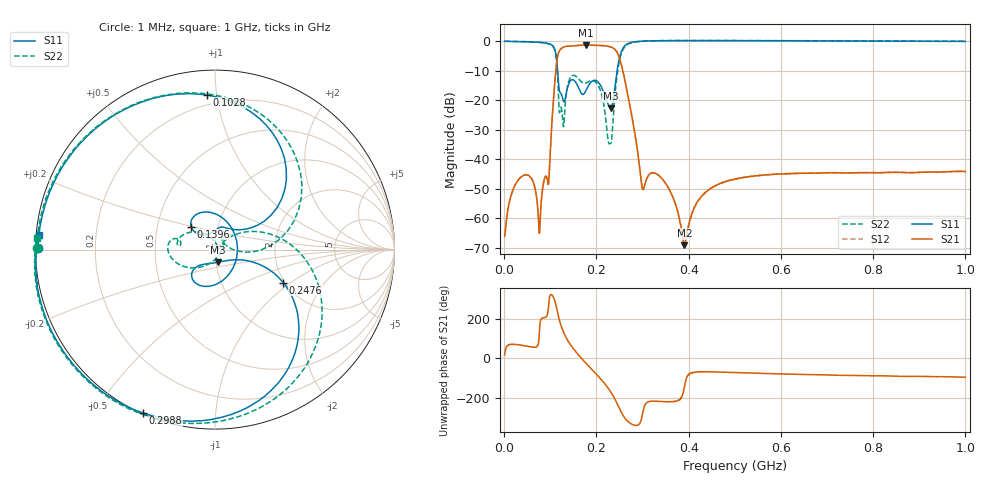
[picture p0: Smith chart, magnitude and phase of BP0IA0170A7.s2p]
!Agilent Technologies,E8358A,US41080443,A.07.50.56
!Agilent E8358A: A.07.50.56
!Date: Tuesday, October 31, 2017 22:14:20
!Correction: S11(Full 2 Port(1,2))
!S21(Full 2 Port(1,2))
!S12(Full 2 Port(1,2))
!S22(Full 2 Port(1,2))
!S2P File: Measurements: S11, S21, S12, S22:
# Hz S  dB  R 50
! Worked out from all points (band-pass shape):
!   1601 points, 1 MHz to 1 GHz, reference 50 ohm
!   highest |S21| = -1.31 dB at 177.7 MHz (marker M1); lowest = -69.2 dB at 390.6 MHz (marker M2)
!   |S21| within 3 dB of the highest: 117.2 MHz to 246.4 MHz (129.2 MHz wide, 71 % of centre)
!   lowest |S11| = -22.8 dB at 231.4 MHz (marker M3), VSWR 1.16, Z = 51.1 - j7.26 ohm
!   |S11| at or under -10 dB: 115.9 MHz to 244.9 MHz (128.9 MHz wide, 71.5 % of centre)
!   |S22| runs from -34.8 to 0.2 dB; largest |S21 - S12| = 0.0046
!   S11 on the Smith chart (normalised r, x): 1 MHz: 0.01, +0.00; 102.8 MHz: 0.14, +0.94; 139.6 MHz: 0.74, +0.20; 247.6 MHz: 1.97, -0.88; 298.8 MHz: 0.00, -0.65; 1 GHz: 0.01, +0.04
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1000000  -0.12 179.6  -66.24 17.8  -65.63 14.7  -0.05 179.5
4.096e7  -0.22 160.7  -45.59 65.4  -45.58 65.8  -0.16 160.7
7.717375e7  -0.46 135.3  -63.59 163.2  -63.59 160.1  -0.43 134.5
9.5905e7  -0.86 109.8  -48.58 -102.8  -48.44 -102.5  -0.91 106.3
1.027731e8  -1.28 93.1  -29.43 -37.5  -29.41 -37.3  -1.40 86.7
1.152606e8  -8.70 31.6  -5.78 -121.4  -5.76 -121.2  -10.19 3.9
1.246262e8  -18.19 79.6  -2.45 157.1  -2.44 157.3  -23.09 49.2
1.396112e8  -14.66 136.1  -1.72 84.2  -1.71 84.3  -13.85 -153.3
1.677081e8  -17.75 21.5  -1.36 0.4  -1.36 0.3  -13.84 165.4
1.776981e8  -16.66 -50.0  -1.31 -25.3  -1.33 -25.4  -14.18 173.2
2.064194e8  -14.38 -133.0  -1.48 -96.1  -1.52 -96.0  -15.82 142.5
2.313944e8  -22.80 -77.2  -2.01 -170.5  -2.02 -170.4  -34.59 -0.6
2.476281e8  -7.48 -25.8  -4.73 118.2  -4.79 118.4  -8.54 9.4
2.701056e8  -0.74 -83.3  -19.85 37.6  -19.87 38.0  -0.91 -70.0
2.988269e8  -0.04 -113.7  -49.41 65.3  -49.40 65.7  -0.05 -107.7
3.344162e8  0.10 -131.3  -45.45 142.5  -45.40 143.5  0.13 -128.1
3.9061e8  0.15 -146.0  -69.24 -149.5  -69.46 -146.5  0.19 -144.3
4.25575e8  0.16 -151.9  -53.03 -68.2  -52.97 -66.8  0.20 -150.6
5.005e8  0.13 -160.5  -46.73 -71.4  -46.77 -71.3  0.17 -159.7
6.672081e8  0.07 -171.9  -44.66 -82.3  -44.77 -82.1  0.11 -171.4
8.339162e8  -0.02 -179.3  -44.51 -88.8  -44.51 -88.8  0.03 -178.5
1e9  -0.13 175.1  -44.19 -94.8  -44.20 -94.9  -0.06 176.1
